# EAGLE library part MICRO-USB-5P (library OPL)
When you use the footprint ,place notice 46 (layer)milling ,there is some important information.
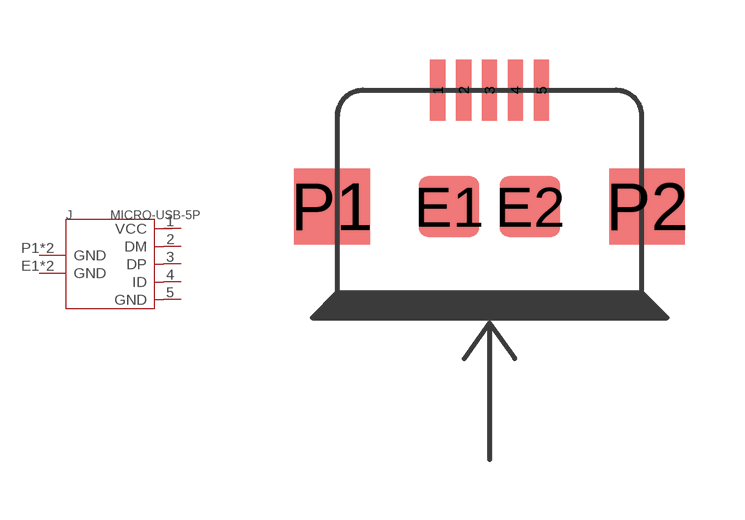
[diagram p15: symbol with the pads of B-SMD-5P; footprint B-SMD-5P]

Designator prefix J

## MICRO-USB-5P-340015001  [B-SMD-5P]
1  VCC
2  DM
3  DP
4  ID
5  GND
E1  GND
E2  GND
P1  GND
P2  GND

## Footprint B-SMD-5P (pad centres in mm)
smd 0.38 x 1.52: 1 -1.3,2.54; 2 -0.65,2.54; 3 0,2.54; 4 0.65,2.54; 5 1.3,2.54
smd 1.524 x 1.524: E1 -1.016,-0.381; E2 1.016,-0.381
smd 1.9 x 1.9: P1 -3.95,-0.381; P2 3.95,-0.381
